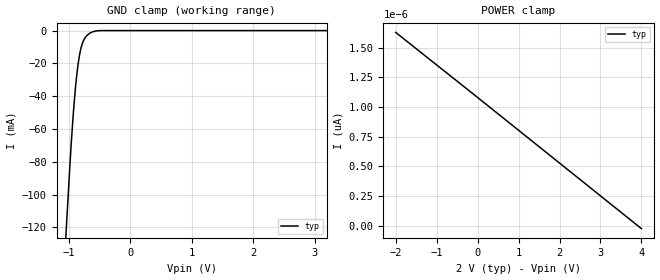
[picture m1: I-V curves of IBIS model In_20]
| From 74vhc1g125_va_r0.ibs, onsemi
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|//////////////////////////////////////////////////////////////////////////////
|//////////////////////////////////////////////////////////////////////////////
[Model]  In_20
Model_type Input
Vinh =  1.50
Vinl =  0.50
|  variable   typ   min   max
C_comp   2.7pF   2.7pF   2.7pF
|//////////////////////////////////////////////////////////////////////////////
[Temperature Range]   25   125   -55
|//////////////////////////////////////////////////////////////////////////////
[Voltage Range]   2.00V   NA   NA
|//////////////////////////////////////////////////////////////////////////////
[POWER Clamp Reference] 2.00V   NA   NA
|//////////////////////////////////////////////////////////////////////////////
[GND Clamp Reference]   0V   NA   NA
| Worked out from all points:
|   GND clamp passes 1 mA (typ) near -0.63 V on its own axis
|//////////////////////////////////////////////////////////////////////////////
[GND Clamp]
|   Voltage   I(typ)   I(min)   I(max)
-2V       -751.7mA   NA         NA
-1.07V    -139.8mA   NA         NA
-1.04V    -120.1mA   NA         NA
-980mV    -80.78mA   NA         NA
-940mV    -57.48mA   NA         NA
-900mV    -38.29mA   NA         NA
-860mV    -23.72mA   NA         NA
-820mV    -13.83mA   NA         NA
-780mV    -7.906mA   NA         NA
-650mV    -1.431mA   NA         NA
-450mV    -8.428uA   NA         NA
4V        1.633pA    NA         NA
|//////////////////////////////////////////////////////////////////////////////
[POWER Clamp]
|   Voltage   I(typ)   I(min)   I(max)
-2V       1.628pA    NA         NA
0V        1.08pA     NA         NA
2V        527.3fA    NA         NA
4V        -25.3fA    NA         NA
